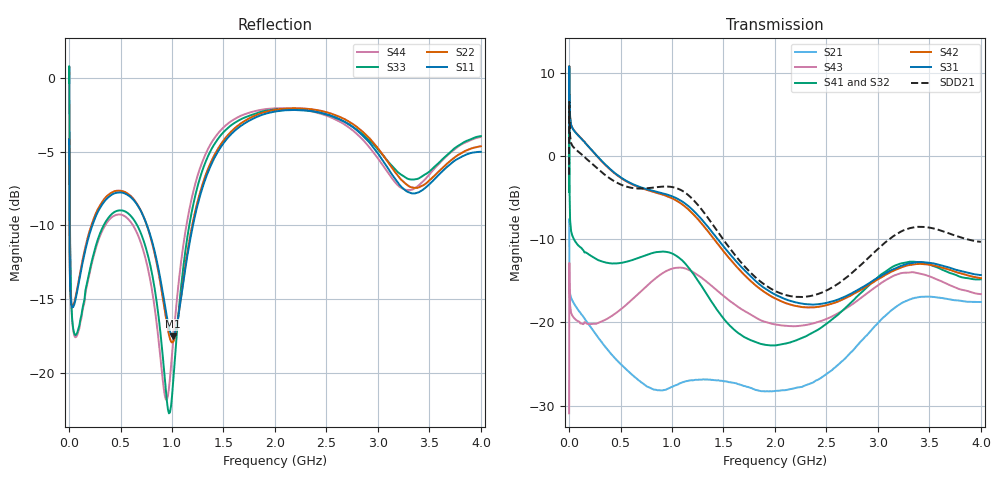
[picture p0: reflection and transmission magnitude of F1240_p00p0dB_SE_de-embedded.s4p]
! Integrated Device Technology
! Corporate Headquarters
! 6024 Silver Creek Valley Road
! San Jose, CA 95138  USA
! Phone:  1-408-284-8200
! Toll Free:  1-800-223-1366
! Webpage:  http://www.idt.com/
! Timing and RF Division
! 515 Groton Road, Suite 102
! Westford, MA 01886-6024
! Device:  F1240
! Description: Dual Intermediate Frequency Digital Variable Gain Amplifier
! Frequency:  10.0 -  500.00 MHz
! Package:  5x5 mm QFN Plastic Package: 32 pin
! Ports:  8 RF, 20 DC
!  Pin  1  = GA3 / Data  Pin 17  = RF OUT_B+
!  Pin  2  = GA4 / CLK  Pin 18  = RF OUT_B-
!  Pin  3  = GA5  Pin 19  = STBY_B
!  Pin  4  = VMODE  Pin 20  = Ground
!  Pin  5  = No Connect  Pin 21  = Ground
!  Pin  6  = GB5  Pin 22  = STB_A
!  Pin  7  = GB4  Pin 23  = RF OUT_A-  = Port 4
!  Pin  8  = GB3  Pin 24  = RF OUT_A+  = Port 3
!  Pin  9  = GB2  Pin 25  = GA0
!  Pin 10  = GB1  Pin 26  = ISET_A
!  Pin 11  = RF IN_B+  Pin 27  = VCC
!  Pin 12  = RF IN_B-  Pin 28  = Ground
!  Pin 13  = Ground  Pin 29  = RF IN_A-  = Port 2
!  Pin 14  = VCC  Pin 30  = RF IN_A+  = Port 1
!  Pin 15  = ISET_B  Pin 31  = GA1
!  Pin 16  = GB0  Pin 32  = GA2 / CSb
! Gain  = +19.5 dB
! State  = 1
! Voltage  = +5.00 V
! Current  = 85.292 mA (one channel only)
! Temperture  =  +25 C
! Test Date  =  2017-10-18
! Board  =  EB4031
! Data:  The device was measured on a custom evaluation board which has
!  individual transmission lines to the RF pins.  Data was collected
!  using a calibrated network analyzer.  The evaluation board was
!  de-embedded using Automatic Fixture Removal.
!  The reference plane is the edge of the package pin.
!  Only Channel A was measured.
!  This data is in single-ended operation.  If your needs are balanced
!  or differential S-parameters then this file needs to be used a
!  linear simulator.
! File Date:  2017-11-10  MJV
! Note:
!  Integrated Device Technology supplies this data as a sample of measured
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# Hz S dB R 100
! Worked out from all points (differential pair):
!   410 points, 500 kHz to 4 GHz, reference 100 ohm
!   strongest paths, dB at 500 kHz, 930 MHz, 1.96 GHz, 2.98 GHz, 4 GHz:
!     S31: 2.8, -4.5, -16.4, -14.7, -14.3
!     S42: 2.8, -4.7, -16.8, -15.0, -14.7
!     S41: -4.3, -11.5, -22.8, -14.8, -14.8
!     S32: -4.3, -11.7, -22.7, -15.2, -15.3
!     S43: -30.9, -13.9, -20.1, -15.7, -16.6
!     S21: -7.9, -28.1, -28.3, -20.3, -17.5
!   taken as a pair (ports 1,2 in; 3,4 out), SDD21 dB: -2.2, -3.6, -15.9, -11.4, -10.3
!   lowest |S11| = -17.5 dB at 1.01 GHz (marker M1), VSWR 1.31, Z = 78.1 - j9.16 ohm
!   |S11| at or under -10 dB: 3.798 MHz to 226.2 MHz (222.4 MHz wide, 193 % of centre); 757.4 MHz to 1.203 GHz (446 MHz wide, 45.5 % of centre)
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500000  -4.49 -5.6  -7.88 -5.8  -29.85 81.1  -37.52 79.1
        -7.88 -5.7  -4.48 -5.5  -37.51 77.8  -29.87 82.3
        2.84 -107.1  -4.27 -108.8  -0.34 0.9  -30.97 -45.4
        -4.29 -107.7  2.83 -105.9  -30.94 -45.7  -0.35 3.2
2500000  -7.22 -43.4  -11.72 -41.8  -19.66 25.0  -29.04 -0.4
         -11.72 -41.9  -7.20 -43.5  -28.99 -0.7  -19.66 25.2
         10.15 177.3  1.72 156.0  -1.08 -56.9  -12.87 -153.0
         1.68 156.1  10.14 177.6  -12.86 -153.0  -1.13 -56.6
4500000  -11.04 -45.5  -15.18 -31.8  -19.81 10.0  -31.81 -14.3
         -15.19 -31.8  -11.02 -45.8  -31.78 -14.5  -19.81 10.1
         7.42 161.6  -3.47 140.1  -5.25 -82.2  -15.22 176.7
         -3.52 140.2  7.42 161.8  -15.20 176.6  -5.30 -82.2
1.7e8  -11.33 -107.1  -19.86 -53.3  -21.96 -44.4  -35.84 -26.1
       -19.88 -53.3  -11.13 -108.5  -35.89 -25.9  -21.97 -44.7
       1.44 116.3  -11.63 85.0  -14.06 -138.7  -20.18 109.1
       -11.61 84.9  1.45 115.6  -20.13 108.8  -14.20 -138.5
5.3e8  -7.80 -164.0  -25.37 -113.8  -23.57 -109.5  -33.65 -75.5
       -25.35 -113.1  -7.70 -165.5  -33.84 -73.4  -23.78 -110.0
       -2.75 23.7  -12.86 -42.3  -9.01 -172.0  -18.29 9.0
       -12.76 -43.5  -2.81 22.4  -18.14 8.9  -9.33 -172.5
1.01e9  -17.53 -154.3  -28.07 -155.9  -22.56 148.2  -30.83 -166.3
        -27.71 -158.4  -17.91 -151.5  -30.83 -160.5  -23.19 147.1
        -4.85 -92.8  -11.95 169.3  -20.74 -118.2  -13.71 -118.3
        -11.74 165.5  -5.10 -95.4  -13.48 -118.3  -17.93 -108.5
4e9  -5.01 -141.1  -17.56 104.8  -23.94 -41.8  -24.93 -25.7
     -17.53 104.7  -4.63 -139.4  -25.84 -10.4  -25.66 -35.0
     -14.29 42.4  -15.30 -61.9  -3.94 -134.2  -18.13 66.5
     -14.80 -75.2  -14.66 48.3  -16.59 57.8  -4.00 -144.0
